|   IBIS model for TI xxx DSP
[IBIS Ver]   5.1
[Disclaimer]   Please be aware that in the absence of a written agreement
|   Texas Instruments(TI) assumes no liability for:
|   (1) The accuracy of the IBIS models provided to your company,
|   however, the IBIS model is compliant to industry standard
|   IQ Level 2a.  Refer to IBIS Quality Section below for
|   for full details.
|   (2) The proper functioning of these Models in your design
|   or for any resulting applications
|   (3) Infringement of patents, copyrights or intellectual
|   property rights resulting from your use of these
|   models.
|   TI provides IBIS Models as a service to our customers and
|   therefore reserves the right to limit distribution of the
|   Models.  The information is subject to change without notice.
[File Name]  sprm771.ibs
[File Rev]   0.1
|   -Initial version
|   -Updated Package model
[Date]   12 Aug 2021
[Source]   Texas Instruments Incorporated
[Copyright]   Property of Texas Instruments Incorporated.
|   Unauthorized reproduction and/or distribution is strictly.
|   prohibited.
|   This product is protected under copyright law and trade
|   secret law as an unpublished work.
|   Created 2012,(C) Copyright 1999-2012,
|   Texas Instruments Incorporated., All Rights Reserved.
|   These commodities are under the U.S. Government
|   distribution license control. As such,they are not to be
|   re-exported without the prior approval of the U.S.
|   Department of Commerce.
[Notes]
  ADC and DAC pins are marked as NC
  XTAL pins are marked as NC
|   Revision History
|   GERNERAL COMMENT: All IBIS Quality Notes below reflect latest release
|   and version of IBIS File
|   File passes ibischk6.0 with 0 errors and 125 warnings
|   Component AM263
[Component] AM263
[Manufacturer] Texas Instruments
[Package Model] AM263_pkg
[Package]
|   typ   min   max
R_pkg   0.11723   0.038857   0.22589
L_pkg   3.378e-9   1.178e-9   5.997e-9
C_pkg   6.073e-13   4.462e-13   1.294e-12
[Pin] Signal_name model_name | Buffer Name
E9   VDD   POWER
E11   VDD   POWER
F9   VDD   POWER
F11   VDD   POWER
G5   VDD   POWER
G6   VDD   POWER
G13   VDD   POWER
G14   VDD   POWER
K5   VDD   POWER
K6   VDD   POWER
K13   VDD   POWER
K14   VDD   POWER
N5   VDD   POWER
N6   VDD   POWER
N13   VDD   POWER
N14   VDD   POWER
R8   VDDA18   POWER
R11   VDDA18   POWER
R6   VDDA18_LDO   POWER
R4   VDDA18_OSC_PLL   POWER
P7   VDDA33   POWER
P9   VDDA33   POWER
P11   VDDA33   POWER
J15   VDDAR1   POWER
D10   VDDAR2   POWER
H3   VDDAR3   POWER
D6   VDDS18   POWER
E15   VDDS18   POWER
L4   VDDS18   POWER
N15   VDDS18   POWER
T3   VDDS18_LDO   POWER
D8   VDDS33   POWER
D12   VDDS33   POWER
H4   VDDS33   POWER
H15   VDDS33   POWER
L15   VDDS33   POWER
P4   VDDS33   POWER
R15   VDDS33   POWER
R9   VDD_F   POWER
J16   VNWA   POWER
N3   VPP   POWER
V15   ADC0_AIN0   NC
U15   ADC0_AIN1   NC
T14   ADC0_AIN2   NC
U14   ADC0_AIN3   NC
U13   ADC0_AIN4   NC
R14   ADC0_AIN5   NC
T11   ADC1_AIN0   NC
U11   ADC1_AIN1   NC
T12   ADC1_AIN2   NC
V12   ADC1_AIN3   NC
U12   ADC1_AIN4   NC
R12   ADC1_AIN5   NC
R10   ADC2_AIN0   NC
T10   ADC2_AIN1   NC
U10   ADC2_AIN2   NC
T9   ADC2_AIN3   NC
V9   ADC2_AIN4   NC
T8   ADC2_AIN5   NC
U7   ADC3_AIN0   NC
U8   ADC3_AIN1   NC
T7   ADC3_AIN2   NC
R7   ADC3_AIN3   NC
V8   ADC3_AIN4   NC
U9   ADC3_AIN5   NC
U6   ADC4_AIN0   NC
V5   ADC4_AIN1   NC
V4   ADC4_AIN2   NC
U5   ADC4_AIN3   NC
V3   ADC4_AIN4   NC
U4   ADC4_AIN5   NC
U16   ADC_CAL0   NC
T15   ADC_CAL1   NC
V14   ADC_VREFHI_G0   NC
V10   ADC_VREFHI_G1   NC
V6   ADC_VREFHI_G2   NC
V13   ADC_VREFLO_G0   NC
V11   ADC_VREFLO_G1   NC
V7   ADC_VREFLO_G2   NC
U3   ATESTV0   NC
V2   ATESTV1   NC
M2   CLKOUT0   bc1833dv40dcpbfbp18ll_ssdlv
T5   DAC_OUT   NC
T13   DAC_VREF0   NC
T6   DAC_VREF1   NC
B2   EPWM0_A   bc1833dv40dcpbfbp18ll_ssdlv
B1   EPWM0_B   bc1833dv40dcpbfbp18ll_ssdlv
D3   EPWM1_A   bc1833dv40dcpbfbp18ll_ssdlv
D2   EPWM1_B   bc1833dv40dcpbfbp18ll_ssdlv
C2   EPWM2_A   bc1833dv40dcpbfbp18ll_ssdlv
C1   EPWM2_B   bc1833dv40dcpbfbp18ll_ssdlv
E2   EPWM3_A   bc1833dv40dcpbfbp18ll_ssdlv
E3   EPWM3_B   bc1833dv40dcpbfbp18ll_ssdlv
D1   EPWM4_A   bc1833dv40dcpbfbp18ll_ssdlv
E4   EPWM4_B   bc1833dv40dcpbfbp18ll_ssdlv
F2   EPWM5_A   bc1833dv40dcpbfbp18ll_ssdlv
G2   EPWM5_B   bc1833dv40dcpbfbp18ll_ssdlv
E1   EPWM6_A   bc1833dv40dcpbfbp18ll_ssdlv
F3   EPWM6_B   bc1833dv40dcpbfbp18ll_ssdlv
F4   EPWM7_A   bc1833dv40dcpbfbp18ll_ssdlv
F1   EPWM7_B   bc1833dv40dcpbfbp18ll_ssdlv
G3   EPWM8_A   bc1833dv40dcpbfbp18ll_ssdlv
H2   EPWM8_B   bc1833dv40dcpbfbp18ll_ssdlv
G1   EPWM9_A   bc1833dv40dcpbfbp18ll_ssdlv
J2   EPWM9_B   bc1833dv40dcpbfbp18ll_ssdlv
G4   EPWM10_A   bc1833dv40dcpbfbp18ll_ssdlv
J3   EPWM10_B   bc1833dv40dcpbfbp18ll_ssdlv
H1   EPWM11_A   bc1833dv40dcpbfbp18ll_ssdlv
J1   EPWM11_B   bc1833dv40dcpbfbp18ll_ssdlv
K2   EPWM12_A   bc1833dv40dcpbfbp18ll_ssdlv
J4   EPWM12_B   bc1833dv40dcpbfbp18ll_ssdlv
K4   EPWM13_A   bc1833dv40dcpbfbp18ll_ssdlv
K3   EPWM13_B   bc1833dv40dcpbfbp18ll_ssdlv
V17   EPWM14_A   bc1833dv40dcpbfbp18ll_ssdlh
T16   EPWM14_B   bc1833dv40dcpbfbp18ll_ssdlh
P15   EPWM15_A   bc1833dv40dcpbfbp18ll_ssdlv
R16   EPWM15_B   bc1833dv40dcpbfbp18ll_ssdlv
B14   EQEP0_A   bc1833dv40dcpbfbp18ll_ssdlh
A14   EQEP0_B   bc1833dv40dcpbfbp18ll_ssdlh
D11   EQEP0_INDEX   bc1833dv40dcpbfbp18ll_ssdlh
C12   EQEP0_STROBE   bc1833dv40dcpbfbp18ll_ssdlh
P2   EXT_REFCLK0   bc1833dv40dcpbfbp18ll_ssdlv
A13   I2C0_SCL   bi2c1833dvfzp18_ssdlh
B13   I2C0_SDA   bi2c1833dvfzp18_ssdlh
D7   I2C1_SCL   bc1833dv40dcpbfbp18ll_ssdlh
C8   I2C1_SDA   bc1833dv40dcpbfbp18ll_ssdlh
A9   LIN1_RXD   bc1833dv40dcpbfbp18ll_ssdlh
B9   LIN1_TXD   bc1833dv40dcpbfbp18ll_ssdlh
B8   LIN2_RXD   bc1833dv40dcpbfbp18ll_ssdlh
A8   LIN2_TXD   bc1833dv40dcpbfbp18ll_ssdlh
M1   MCAN0_RX   bc1833dv40dcpbfbp18ll_ssdlv
L1   MCAN0_TX   bc1833dv40dcpbfbp18ll_ssdlv
L2   MCAN1_RX   bc1833dv40dcpbfbp18ll_ssdlv
K1   MCAN1_TX   bc1833dv40dcpbfbp18ll_ssdlv
A12   MCAN2_RX   bc1833dv40dcpbfbp18ll_ssdlh
B12   MCAN2_TX   bc1833dv40dcpbfbp18ll_ssdlh
M17   MDIO0_MDC   bc1833dv40dcpbfbp18ll_ssdlv
N16   MDIO0_MDIO   bc1833dv40dcpbfbp18ll_ssdlv
A5   MMC0_CD   bc1833dv40dcpbfbp18ll_ssdlh
B6   MMC0_CLK   bc1833dv40dcpbfbp18ll_ssdlh
A4   MMC0_CMD   bc1833dv40dcpbfbp18ll_ssdlh
B5   MMC0_D0   bc1833dv40dcpbfbp18ll_ssdlh
B4   MMC0_D1   bc1833dv40dcpbfbp18ll_ssdlh
A3   MMC0_D2   bc1833dv40dcpbfbp18ll_ssdlh
A2   MMC0_D3   bc1833dv40dcpbfbp18ll_ssdlh
C6   MMC0_WP   bc1833dv40dcpbfbp18ll_ssdlh
R2   PORZ   ihhv1833dvhyp18ll_ssdhv
L18   PR0_MDIO0_MDC   bc1833dv40dcpbfbp18ll_ssdlv
L17   PR0_MDIO0_MDIO   bc1833dv40dcpbfbp18ll_ssdlv
K17   PR0_PRU0_GPO0   bc1833dv40dcpbfbp18ll_ssdlv
K18   PR0_PRU0_GPO1   bc1833dv40dcpbfbp18ll_ssdlv
J18   PR0_PRU0_GPO2   bc1833dv40dcpbfbp18ll_ssdlv
J17   PR0_PRU0_GPO3   bc1833dv40dcpbfbp18ll_ssdlv
K16   PR0_PRU0_GPO4   bc1833dv40dcpbfbp18ll_ssdlv
G17   PR0_PRU0_GPO5   bc1833dv40dcpbfbp18ll_ssdlv
K15   PR0_PRU0_GPO6   bc1833dv40dcpbfbp18ll_ssdlv
G15   PR0_PRU0_GPO8   bc1833dv40dcpbfbp18ll_ssdlv
F17   PR0_PRU0_GPO9   bc1833dv40dcpbfbp18ll_ssdlv
G18   PR0_PRU0_GPO10   bc1833dv40dcpbfbp18ll_ssdlv
M16   PR0_PRU0_GPO11   bc1833dv40dcpbfbp18ll_ssdlv
M15   PR0_PRU0_GPO12   bc1833dv40dcpbfbp18ll_ssdlv
H17   PR0_PRU0_GPO13   bc1833dv40dcpbfbp18ll_ssdlv
H16   PR0_PRU0_GPO14   bc1833dv40dcpbfbp18ll_ssdlv
L16   PR0_PRU0_GPO15   bc1833dv40dcpbfbp18ll_ssdlv
H18   PR0_PRU0_GPO16   bc1833dv40dcpbfbp18ll_ssdlv
F18   PR0_PRU1_GPO0   bc1833dv40dcpbfbp18ll_ssdlv
G16   PR0_PRU1_GPO1   bc1833dv40dcpbfbp18ll_ssdlv
E17   PR0_PRU1_GPO2   bc1833dv40dcpbfbp18ll_ssdlv
E18   PR0_PRU1_GPO3   bc1833dv40dcpbfbp18ll_ssdlv
F16   PR0_PRU1_GPO4   bc1833dv40dcpbfbp18ll_ssdlv
F15   PR0_PRU1_GPO5   bc1833dv40dcpbfbp18ll_ssdlv
E16   PR0_PRU1_GPO6   bc1833dv40dcpbfbp18ll_ssdlv
D18   PR0_PRU1_GPO8   bc1833dv40dcpbfbp18ll_ssdlv
C18   PR0_PRU1_GPO9   bc1833dv40dcpbfbp18ll_ssdlv
D17   PR0_PRU1_GPO10   bc1833dv40dcpbfbp18ll_ssdlv
B18   PR0_PRU1_GPO11   bc1833dv40dcpbfbp18ll_ssdlv
B17   PR0_PRU1_GPO12   bc1833dv40dcpbfbp18ll_ssdlv
D16   PR0_PRU1_GPO13   bc1833dv40dcpbfbp18ll_ssdlv
C17   PR0_PRU1_GPO14   bc1833dv40dcpbfbp18ll_ssdlv
A17   PR0_PRU1_GPO15   bc1833dv40dcpbfbp18ll_ssdlv
C16   PR0_PRU1_GPO16   bc1833dv40dcpbfbp18ll_ssdlv
C15   PR0_PRU1_GPO18   bc1833dv40dcpbfbp18ll_ssdlv
D15   PR0_PRU1_GPO19   bc1833dv40dcpbfbp18ll_ssdlv
N2   QSPI0_CLK   bc1833dv40dcpbfbp18ll_ssdlv
P1   QSPI0_CSN0   bc1833dv40dcpbfbp18ll_ssdlv
R3   QSPI0_CSN1   bc1833dv40dcpbfbp18ll_ssdlv
N1   QSPI0_D0   bc1833dv40dcpbfbp18ll_ssdlv
N4   QSPI0_D1   bc1833dv40dcpbfbp18ll_ssdlv
M4   QSPI0_D2   bc1833dv40dcpbfbp18ll_ssdlv
P3   QSPI0_D3   bc1833dv40dcpbfbp18ll_ssdlv
U17   RGMII1_RD0   bc1833dv40dcpbfbp18ll_ssdlv
T17   RGMII1_RD1   bc1833dv40dcpbfbp18ll_ssdlv
U18   RGMII1_RD2   bc1833dv40dcpbfbp18ll_ssdlv
T18   RGMII1_RD3   bc1833dv40dcpbfbp18ll_ssdlv
R17   RGMII1_RXC   bc1833dv40dcpbfbp18ll_ssdlv
R18   RGMII1_RX_CTL   bc1833dv40dcpbfbp18ll_ssdlv
P16   RGMII1_TD0   bc1833dv40dcpbfbp18ll_ssdlv
P17   RGMII1_TD1   bc1833dv40dcpbfbp18ll_ssdlv
P18   RGMII1_TD2   bc1833dv40dcpbfbp18ll_ssdlv
N17   RGMII1_TD3   bc1833dv40dcpbfbp18ll_ssdlv
N18   RGMII1_TXC   bc1833dv40dcpbfbp18ll_ssdlv
M18   RGMII1_TX_CTL   bc1833dv40dcpbfbp18ll_ssdlv
D4   SAFETY_ERRORN   bc1833dv40dcpbfbp18ll_ssdlv
B16   SDFM0_CLK0   bc1833dv40dcpbfbp18ll_ssdlh
A16   SDFM0_CLK1   bc1833dv40dcpbfbp18ll_ssdlh
B15   SDFM0_CLK2   bc1833dv40dcpbfbp18ll_ssdlh
A15   SDFM0_CLK3   bc1833dv40dcpbfbp18ll_ssdlh
D14   SDFM0_D0   bc1833dv40dcpbfbp18ll_ssdlh
D13   SDFM0_D1   bc1833dv40dcpbfbp18ll_ssdlh
C13   SDFM0_D2   bc1833dv40dcpbfbp18ll_ssdlh
C14   SDFM0_D3   bc1833dv40dcpbfbp18ll_ssdlh
A11   SPI0_CLK   bc1833dv40dcpbfbp18ll_ssdlh
C11   SPI0_CS0   bc1833dv40dcpbfbp18ll_ssdlh
C10   SPI0_D0   bc1833dv40dcpbfbp18ll_ssdlh
B11   SPI0_D1   bc1833dv40dcpbfbp18ll_ssdlh
A10   SPI1_CLK   bc1833dv40dcpbfbp18ll_ssdlh
C9   SPI1_CS0   bc1833dv40dcpbfbp18ll_ssdlh
B10   SPI1_D0   bc1833dv40dcpbfbp18ll_ssdlh
D9   SPI1_D1   bc1833dv40dcpbfbp18ll_ssdlh
B3   TCK   iq1833dvtckpbfbp18ll_ssdhh
C5   TDI   bc1833dv40dcpbfbp18ll_ssdlh
C4   TDO   bc1833dv40dcpbfbp18ll_ssdlh
U1   TEMPCAL   NC
D5   TMS   bc1833dv40dcpbfbp18ll_ssdlh
B7   UART0_CTSN   bc1833dv40dcpbfbp18ll_ssdlh
C7   UART0_RTSN   bc1833dv40dcpbfbp18ll_ssdlh
A7   UART0_RXD   bc1833dv40dcpbfbp18ll_ssdlh
A6   UART0_TXD   bc1833dv40dcpbfbp18ll_ssdlh
L3   UART1_RXD   bc1833dv40dcpbfbp18ll_ssdlv
M3   UART1_TXD   bc1833dv40dcpbfbp18ll_ssdlv
T4   VDD_TEMP   NC
U2   VSYS_MON   NC
C3   WARMRSTN   bc1833dv40dcpbfbp18ll_od_fs_ssdlv
T1   XTAL_XI   NC
R1   XTAL_XO   NC
A1   VSS   GND
A18   VSS   GND
E5   VSS   GND
E6   VSS   GND
E7   VSS   GND
E8   VSS   GND
E10   VSS   GND
E12   VSS   GND
E13   VSS   GND
E14   VSS   GND
F5   VSS   GND
F6   VSS   GND
F7   VSS   GND
F8   VSS   GND
F10   VSS   GND
F12   VSS   GND
F13   VSS   GND
F14   VSS   GND
G7   VSS   GND
G8   VSS   GND
G9   VSS   GND
G10   VSS   GND
G11   VSS   GND
G12   VSS   GND
H5   VSS   GND
H6   VSS   GND
H7   VSS   GND
H8   VSS   GND
H9   VSS   GND
H10   VSS   GND
H11   VSS   GND
H12   VSS   GND
H13   VSS   GND
H14   VSS   GND
J5   VSS   GND
J6   VSS   GND
J7   VSS   GND
J8   VSS   GND
J9   VSS   GND
J10   VSS   GND
J11   VSS   GND
J12   VSS   GND
J13   VSS   GND
J14   VSS   GND
K7   VSS   GND
K8   VSS   GND
K9   VSS   GND
K10   VSS   GND
K11   VSS   GND
K12   VSS   GND
L5   VSS   GND
L6   VSS   GND
L7   VSS   GND
L8   VSS   GND
L9   VSS   GND
L10   VSS   GND
L11   VSS   GND
L12   VSS   GND
L13   VSS   GND
L14   VSS   GND
M5   VSS   GND
M6   VSS   GND
M7   VSS   GND
M8   VSS   GND
M9   VSS   GND
M10   VSS   GND
M11   VSS   GND
M12   VSS   GND
M13   VSS   GND
M14   VSS   GND
N7   VSS   GND
N8   VSS   GND
N9   VSS   GND
N10   VSS   GND
N11   VSS   GND
N12   VSS   GND
P5   VSS   GND
P13   VSS   GND
P14   VSS   GND
T2   VSS   GND
V18   VSS   GND
P6   VSSA   GND
P8   VSSA   GND
P10   VSSA   GND
P12   VSSA   GND
R5   VSSA   GND
R13   VSSA   GND
V1   VSSA   GND
V16   VSSA   GND
|   BC1833DV40DCPBFBP18LL_SSDLH
[Model Selector] bc1833dv40dcpbfbp18ll_ssdlh
|SC1 IS A SLEW RATE CONTROL PIN
|5% SUPPLY VARIATION MODES WITH 1.8V NOM SUPPLY
BC40D_H_PUPDOFF_5P_SC1_1P8  Cell operated at 1.8(nom)
|BC40D_H_PUPDOFF_5P_SC1_1P8; BUFFER WITH WEAK PULUP/PULLDOWN OFF AT 5% SUPPLY
|VARIATION WITH SC1=1 MEANING SLOW MODE OF OPERATION
BC40D_H_PD_ON_5P_!SC1_1P8  Cell operated at 1.8(nom)
|BC40D_H_PD_ON_5P_!SC1_1P8; BUFFER WITH WEAK_PULLDOWN_ON AT 5% SUPPLY
|VARIATION WITH SC1=0 MEANING FAST MODE OF OPERATION
BC40D_H_PD_ON_5P_SC1_1P8  Cell operated at 1.8(nom)
|BC40D_H_PD_ON_5P_SC1_1P8; BUFFER WITH WEAK_PULLDOWN_ON AT 5% SUPPLY
|VARIATION WITH SC1=1 MEANING SLOW MODE OF OPERATION
BC40D_H_PU_ON_5P_!SC1_1P8  Cell operated at 1.8(nom)
|BC40D_H_PU_ON_5P_!SC1_1P8; BUFFER WITH WEAK_PULLUP_ON AT 5% SUPPLY
|VARIATION WITH SC1=0 MEANING FAST MODE OF OPERATION
BC40D_H_PUPDOFF_5P_!SC1_1P8  Cell operated at 1.8(nom)
|BC40D_H_PUPDOFF_5P_!SC1_1P8; BUFFER WITH WEAK PULUP/PULLDOWN OFF AT 5% SUPPLY
|VARIATION WITH SC1=0 MEANING FAST MODE OF OPERATION
BC40D_H_PU_ON_5P_SC1_1P8  Cell operated at 1.8(nom)
|BC40D_H_PU_ON_5P_SC1_1P8; BUFFER WITH WEAK_PULLUP_ON AT 5% SUPPLY
|VARIATION WITH SC1=1 MEANING SLOW MODE OF OPERATION
|5% SUPPLY VARIATION MODES WITH 3.3V NOM SUPPLY
BC40D_H_PUPDOFF_5P_SC1_3P3  Cell operated at 3.3(nom)
|BC40D_H_PUPDOFF_5P_SC1_3P3; BUFFER WITH WEAK PULUP/PULLDOWN OFF AT 5% SUPPLY
|VARIATION WITH SC1=1 MEANING SLOW MODE OF OPERATION
BC40D_H_PD_ON_5P_!SC1_3P3  Cell operated at 3.3(nom)
|BC40D_H_PD_ON_5P_!SC1_3P3; BUFFER WITH WEAK_PULLDOWN_ON AT 5% SUPPLY
|VARIATION WITH SC1=0 MEANING FAST MODE OF OPERATION
BC40D_H_PD_ON_5P_SC1_3P3  Cell operated at 3.3(nom)
|BC40D_H_PD_ON_5P_SC1_3P3; BUFFER WITH WEAK_PULLDOWN_ON AT 5% SUPPLY
|VARIATION WITH SC1=1 MEANING SLOW MODE OF OPERATION
BC40D_H_PU_ON_5P_!SC1_3P3  Cell operated at 3.3(nom)
|BC40D_H_PU_ON_5P_!SC1_3P3; BUFFER WITH WEAK_PULLUP_ON AT 5% SUPPLY
|VARIATION WITH SC1=0 MEANING FAST MODE OF OPERATION
BC40D_H_PUPDOFF_5P_!SC1_3P3  Cell operated at 3.3(nom)
|BC40D_H_PUPDOFF_5P_!SC1_3P3; BUFFER WITH WEAK PULUP/PULLDOWN OFF AT 5% SUPPLY
|VARIATION WITH SC1=0 MEANING FAST MODE OF OPERATION
BC40D_H_PU_ON_5P_SC1_3P3  Cell operated at 3.3(nom)
|BC40D_H_PU_ON_5P_SC1_3P3; BUFFER WITH WEAK_PULLUP_ON AT 5% SUPPLY
|VARIATION WITH SC1=1 MEANING SLOW MODE OF OPERATION
| 10% SUPPLY VARIATION MODES WITH 1.8V NOM SUPPLY
BC40D_H_PUPDOFF_10P_SC1_1P8  Cell operated at 1.8(nom)
|BC40D_H_PUPDOFF_10P_SC1_1P8; BUFFER WITH WEAK PULUP/PULLDOWN OFF AT 10% SUPPLY
|VARIATION WITH SC1=1 MEANING SLOW MODE OF OPERATION
BC40D_H_PD_ON_10P_!SC1_1P8  Cell operated at 1.8(nom)
|BC40D_H_PD_ON_10P_!SC1_1P8; BUFFER WITH WEAK_PULLDOWN_ON AT 10% SUPPLY
|VARIATION WITH SC1=0 MEANING FAST MODE OF OPERATION
BC40D_H_PD_ON_10P_SC1_1P8  Cell operated at 1.8(nom)
|BC40D_H_PD_ON_10P_SC1_1P8; BUFFER WITH WEAK_PULLDOWN_ON AT 10% SUPPLY
|VARIATION WITH SC1=1 MEANING SLOW MODE OF OPERATION
BC40D_H_PU_ON_10P_!SC1_1P8  Cell operated at 1.8(nom)
|BC40D_H_PU_ON_10P_!SC1_1P8; BUFFER WITH WEAK_PULLUP_ON AT 10% SUPPLY
|VARIATION WITH SC1=0 MEANING FAST MODE OF OPERATION
BC40D_H_PUPDOFF_10P_!SC1_1P8  Cell operated at 1.8(nom)
|BC40D_H_PUPDOFF_10P_!SC1_1P8; BUFFER WITH WEAK PULUP/PULLDOWN OFF AT 10% SUPPLY
|VARIATION WITH SC1=0 MEANING FAST MODE OF OPERATION
BC40D_H_PU_ON_10P_SC1_1P8  Cell operated at 1.8(nom)
|BC40D_H_PU_ON_10P_SC1_1P8; BUFFER WITH WEAK_PULLUP_ON AT 10% SUPPLY
|VARIATION WITH SC1=1 MEANING SLOW MODE OF OPERATION
| 10% SUPPLY VARIATION MODES WITH 3.3V NOM SUPPLY
BC40D_H_PUPDOFF_10P_SC1_3P3  Cell operated at 3.3(nom)
|BC40D_H_PUPDOFF_10P_SC1_3P3; BUFFER WITH WEAK PULUP/PULLDOWN OFF AT 10% SUPPLY
|VARIATION WITH SC1=1 MEANING SLOW MODE OF OPERATION
BC40D_H_PD_ON_10P_!SC1_3P3  Cell operated at 3.3(nom)
|BC40D_H_PD_ON_10P_!SC1_3P3; BUFFER WITH WEAK_PULLDOWN_ON 10% SUPPLY
|VARIATION WITH SC1=0 MEANING FAST MODE OF OPERATION
BC40D_H_PD_ON_10P_SC1_3P3  Cell operated at 3.3(nom)
|BC40D_H_PD_ON_10P_SC1_3P3; BUFFER WITH WEAK_PULLDOWN_ON AT 10% SUPPLY
|VARIATION WITH SC1=1 MEANING SLOW MODE OF OPERATION
BC40D_H_PU_ON_10P_!SC1_3P3  Cell operated at 3.3(nom)
|BC40D_H_PU_ON_10P_!SC1_3P3; BUFFER WITH WEAK_PULLUP_ON AT 10% SUPPLY
|VARIATION WITH SC1=0 MEANING FAST MODE OF OPERATION
BC40D_H_PUPDOFF_10P_!SC1_3P3  Cell operated at 3.3(nom)
|BC40D_H_PUPDOFF_10P_!SC1_3P3; BUFFER WITH WEAK PULUP/PULLDOWN OFF AT 10% SUPPLY
|VARIATION WITH SC1=0 MEANING FAST MODE OF OPERATION
BC40D_H_PU_ON_10P_SC1_3P3  Cell operated at 3.3(nom)
|BC40D_H_PU_ON_10P_SC1_3P3; BUFFER WITH WEAK_PULLUP_ON AT 10% SUPPLY
|VARIATION WITH SC1=1 MEANING SLOW MODE OF OPERATION
|   BC1833DV40DCPBFBP18LL_SSDLV
[Model Selector] bc1833dv40dcpbfbp18ll_ssdlv
|SC1 IS A SLEW RATE CONTROL PIN
|5% SUPPLY VARIATION MODES WITH 1.8V NOM SUPPLY
BC40D_V_PUPDOFF_5P_SC1_1P8  Cell operated at 1.8(nom)
|BC40D_V_PUPDOFF_5P_SC1_1P8; BUFFER WITH WEAK PULUP/PULLDOWN OFF AT 5% SUPPLY
|VARIATION WITH SC1=1 MEANING SLOW MODE OF OPERATION
BC40D_V_PD_ON_5P_!SC1_1P8  Cell operated at 1.8(nom)
|BC40D_V_PD_ON_5P_!SC1_1P8; BUFFER WITH WEAK_PULLDOWN_ON AT 5% SUPPLY
|VARIATION WITH SC1=0 MEANING FAST MODE OF OPERATION
BC40D_V_PD_ON_5P_SC1_1P8  Cell operated at 1.8(nom)
|BC40D_V_PD_ON_5P_SC1_1P8; BUFFER WITH WEAK_PULLDOWN_ON AT 5% SUPPLY
|VARIATION WITH SC1=1 MEANING SLOW MODE OF OPERATION
BC40D_V_PU_ON_5P_!SC1_1P8  Cell operated at 1.8(nom)
|BC40D_V_PU_ON_5P_!SC1_1P8; BUFFER WITH WEAK_PULLUP_ON AT 5% SUPPLY
|VARIATION WITH SC1=0 MEANING FAST MODE OF OPERATION
BC40D_V_PUPDOFF_5P_!SC1_1P8  Cell operated at 1.8(nom)
|BC40D_V_PUPDOFF_5P_!SC1_1P8; BUFFER WITH WEAK PULUP/PULLDOWN OFF AT 5% SUPPLY
|VARIATION WITH SC1=0 MEANING FAST MODE OF OPERATION
BC40D_V_PU_ON_5P_SC1_1P8  Cell operated at 1.8(nom)
|BC40D_V_PU_ON_5P_SC1_1P8; BUFFER WITH WEAK_PULLUP_ON AT 5% SUPPLY
|VARIATION WITH SC1=1 MEANING SLOW MODE OF OPERATION
|5% SUPPLY VARIATION MODES WITH 3.3V NOM SUPPLY
BC40D_V_PUPDOFF_5P_SC1_3P3  Cell operated at 3.3(nom)
|BC40D_V_PUPDOFF_5P_SC1_3P3; BUFFER WITH WEAK PULUP/PULLDOWN OFF AT 5% SUPPLY
|VARIATION WITH SC1=1 MEANING SLOW MODE OF OPERATION
BC40D_V_PD_ON_5P_!SC1_3P3  Cell operated at 3.3(nom)
|BC40D_V_PD_ON_5P_!SC1_3P3; BUFFER WITH WEAK_PULLDOWN_ON AT 5% SUPPLY
|VARIATION WITH SC1=0 MEANING FAST MODE OF OPERATION
BC40D_V_PD_ON_5P_SC1_3P3  Cell operated at 3.3(nom)
|BC40D_V_PD_ON_5P_SC1_3P3; BUFFER WITH WEAK_PULLDOWN_ON AT 5% SUPPLY
|VARIATION WITH SC1=1 MEANING SLOW MODE OF OPERATION
BC40D_V_PU_ON_5P_!SC1_3P3  Cell operated at 3.3(nom)
|BC40D_V_PU_ON_5P_!SC1_3P3; BUFFER WITH WEAK_PULLUP_ON AT 5% SUPPLY
|VARIATION WITH SC1=0 MEANING FAST MODE OF OPERATION
BC40D_V_PUPDOFF_5P_!SC1_3P3  Cell operated at 3.3(nom)
|BC40D_V_PUPDOFF_5P_!SC1_3P3; BUFFER WITH WEAK PULUP/PULLDOWN OFF AT 5% SUPPLY
|VARIATION WITH SC1=0 MEANING FAST MODE OF OPERATION
BC40D_V_PU_ON_5P_SC1_3P3  Cell operated at 3.3(nom)
|BC40D_V_PU_ON_5P_SC1_3P3; BUFFER WITH WEAK_PULLUP_ON AT 5% SUPPLY
|VARIATION WITH SC1=1 MEANING SLOW MODE OF OPERATION
| 10% SUPPLY VARIATION MODES WITH 1.8V NOM SUPPLY
BC40D_V_PUPDOFF_10P_SC1_1P8  Cell operated at 1.8(nom)
|BC40D_V_PUPDOFF_10P_SC1_1P8; BUFFER WITH WEAK PULUP/PULLDOWN OFF AT 10% SUPPLY
|VARIATION WITH SC1=1 MEANING SLOW MODE OF OPERATION
BC40D_V_PD_ON_10P_!SC1_1P8  Cell operated at 1.8(nom)
|BC40D_V_PD_ON_10P_!SC1_1P8; BUFFER WITH WEAK_PULLDOWN_ON AT 10% SUPPLY
|VARIATION WITH SC1=0 MEANING FAST MODE OF OPERATION
BC40D_V_PD_ON_10P_SC1_1P8  Cell operated at 1.8(nom)
|BC40D_V_PD_ON_10P_SC1_1P8; BUFFER WITH WEAK_PULLDOWN_ON AT 10% SUPPLY
|VARIATION WITH SC1=1 MEANING SLOW MODE OF OPERATION
BC40D_V_PU_ON_10P_!SC1_1P8  Cell operated at 1.8(nom)
|BC40D_V_PU_ON_10P_!SC1_1P8; BUFFER WITH WEAK_PULLUP_ON AT 10% SUPPLY
|VARIATION WITH SC1=0 MEANING FAST MODE OF OPERATION
BC40D_V_PUPDOFF_10P_!SC1_1P8  Cell operated at 1.8(nom)
|BC40D_V_PUPDOFF_10P_!SC1_1P8; BUFFER WITH WEAK PULUP/PULLDOWN OFF AT 10% SUPPLY
|VARIATION WITH SC1=0 MEANING FAST MODE OF OPERATION
BC40D_V_PU_ON_10P_SC1_1P8  Cell operated at 1.8(nom)
|BC40D_V_PU_ON_10P_SC1_1P8; BUFFER WITH WEAK_PULLUP_ON AT 10% SUPPLY
|VARIATION WITH SC1=1 MEANING SLOW MODE OF OPERATION
| 10% SUPPLY VARIATION MODES WITH 3.3V NOM SUPPLY
BC40D_V_PUPDOFF_10P_SC1_3P3  Cell operated at 3.3(nom)
|BC40D_V_PUPDOFF_10P_SC1_3P3; BUFFER WITH WEAK PULUP/PULLDOWN OFF AT 10% SUPPLY
|VARIATION WITH SC1=1 MEANING SLOW MODE OF OPERATION
BC40D_V_PD_ON_10P_!SC1_3P3  Cell operated at 3.3(nom)
|BC40D_V_PD_ON_10P_!SC1_3P3; BUFFER WITH WEAK_PULLDOWN_ON 10% SUPPLY
|VARIATION WITH SC1=0 MEANING FAST MODE OF OPERATION
BC40D_V_PD_ON_10P_SC1_3P3  Cell operated at 3.3(nom)
|BC40D_V_PD_ON_10P_SC1_3P3; BUFFER WITH WEAK_PULLDOWN_ON AT 10% SUPPLY
|VARIATION WITH SC1=1 MEANING SLOW MODE OF OPERATION
BC40D_V_PU_ON_10P_!SC1_3P3  Cell operated at 3.3(nom)
|BC40D_V_PU_ON_10P_!SC1_3P3; BUFFER WITH WEAK_PULLUP_ON AT 10% SUPPLY
|VARIATION WITH SC1=0 MEANING FAST MODE OF OPERATION
BC40D_V_PUPDOFF_10P_!SC1_3P3  Cell operated at 3.3(nom)
|BC40D_V_PUPDOFF_10P_!SC1_3P3; BUFFER WITH WEAK PULUP/PULLDOWN OFF AT 10% SUPPLY
|VARIATION WITH SC1=0 MEANING FAST MODE OF OPERATION
BC40D_V_PU_ON_10P_SC1_3P3  Cell operated at 3.3(nom)
|BC40D_V_PU_ON_10P_SC1_3P3; BUFFER WITH WEAK_PULLUP_ON AT 10% SUPPLY
|VARIATION WITH SC1=1 MEANING SLOW MODE OF OPERATION
|   BI2C1833DVFZP18_SSDLH
[Model Selector] bi2c1833dvfzp18_ssdlh
BI2C1833_NORAML_5P_1P8  Cell operated at 1.8(nom)
|BI2C1833_NORAML_5P_1P8; I2C MODE AT 1.8V WITH 5% SUPPLY VARIATION
BI2C1833_NORAML_5P_3P3  Cell operated at 3.3(nom)
|BI2C1833_NORAML_5P_3P3; I2C MODE AT 3.3V WITH 5% SUPPLY VARIATION
BI2C1833_NORAML_10P_1P8  Cell operated at 1.8(nom)
|BI2C1833_NORAML_10P_1P8; I2C MODE AT 1.8V WITH 10% SUPPLY VARIATION
BI2C1833_NORAML_10P_3P3  Cell operated at 3.3(nom)
|BI2C1833_NORAML_10P_3P3; I2C MODE AT 3.3V WITH 10% SUPPLY VARIATION
|   IHHV1833DVHYP18LL_SSDHV
[Model Selector] ihhv1833dvhyp18ll_ssdhv
IHHV_NORAML_5P_1P8  Cell operated at 1.8(nom)
|IHHV_NORAML_5P_1P8; NORMAL MODE AT 1.8V WITH 5% SUPPLY VARIATION
IHHV_NORAML_5P_3P3  Cell operated at 3.3(nom)
|IHHV_NORAML_5P_3P3; NORMAL MODE AT 3.3V WITH 5% SUPPLY VARIATION
IHHV_NORAML_10P_1P8  Cell operated at 1.8(nom)
|IHHV_NORAML_10P_1P8; NORMAL MODE AT 1.8V WITH 10% SUPPLY VARIATION
IHHV_NORAML_10P_3P3  Cell operated at 3.3(nom)
|IHHV_NORAML_10P_3P3; NORMAL MODE AT 3.3V WITH 10% SUPPLY VARIATION
|   BC1833DV40DCPBFBP18LL_OD_FS_SSDLV
[Model Selector] bc1833dv40dcpbfbp18ll_od_fs_ssdlv
|SC1 IS A SLEW RATE CONTROL PIN
|5% SUPPLY VARIATION MODES WITH 1.8V NOM SUPPLY
BC40D_V_PUPDOFF_5P_SC1_1P8  Cell operated at 1.8(nom)
|BC40D_V_PUPDOFF_5P_SC1_1P8; BUFFER WITH WEAK PULUP/PULLDOWN OFF AT 5% SUPPLY
|VARIATION WITH SC1=1 MEANING SLOW MODE OF OPERATION
BC40D_V_PD_ON_5P_!SC1_1P8  Cell operated at 1.8(nom)
|BC40D_V_PD_ON_5P_!SC1_1P8; BUFFER WITH WEAK_PULLDOWN_ON AT 5% SUPPLY
|VARIATION WITH SC1=0 MEANING FAST MODE OF OPERATION
BC40D_V_PD_ON_5P_SC1_1P8  Cell operated at 1.8(nom)
|BC40D_V_PD_ON_5P_SC1_1P8; BUFFER WITH WEAK_PULLDOWN_ON AT 5% SUPPLY
|VARIATION WITH SC1=1 MEANING SLOW MODE OF OPERATION
BC40D_V_PU_ON_5P_!SC1_1P8  Cell operated at 1.8(nom)
|BC40D_V_PU_ON_5P_!SC1_1P8; BUFFER WITH WEAK_PULLUP_ON AT 5% SUPPLY
|VARIATION WITH SC1=0 MEANING FAST MODE OF OPERATION
BC40D_V_PUPDOFF_5P_!SC1_1P8  Cell operated at 1.8(nom)
|BC40D_V_PUPDOFF_5P_!SC1_1P8; BUFFER WITH WEAK PULUP/PULLDOWN OFF AT 5% SUPPLY
|VARIATION WITH SC1=0 MEANING FAST MODE OF OPERATION
BC40D_V_PU_ON_5P_SC1_1P8  Cell operated at 1.8(nom)
|BC40D_V_PU_ON_5P_SC1_1P8; BUFFER WITH WEAK_PULLUP_ON AT 5% SUPPLY
|VARIATION WITH SC1=1 MEANING SLOW MODE OF OPERATION
|5% SUPPLY VARIATION MODES WITH 3.3V NOM SUPPLY
BC40D_V_PUPDOFF_5P_SC1_3P3  Cell operated at 3.3(nom)
|BC40D_V_PUPDOFF_5P_SC1_3P3; BUFFER WITH WEAK PULUP/PULLDOWN OFF AT 5% SUPPLY
|VARIATION WITH SC1=1 MEANING SLOW MODE OF OPERATION
BC40D_V_PD_ON_5P_!SC1_3P3  Cell operated at 3.3(nom)
|BC40D_V_PD_ON_5P_!SC1_3P3; BUFFER WITH WEAK_PULLDOWN_ON AT 5% SUPPLY
|VARIATION WITH SC1=0 MEANING FAST MODE OF OPERATION
BC40D_V_PD_ON_5P_SC1_3P3  Cell operated at 3.3(nom)
|BC40D_V_PD_ON_5P_SC1_3P3; BUFFER WITH WEAK_PULLDOWN_ON AT 5% SUPPLY
|VARIATION WITH SC1=1 MEANING SLOW MODE OF OPERATION
BC40D_V_PU_ON_5P_!SC1_3P3  Cell operated at 3.3(nom)
|BC40D_V_PU_ON_5P_!SC1_3P3; BUFFER WITH WEAK_PULLUP_ON AT 5% SUPPLY
|VARIATION WITH SC1=0 MEANING FAST MODE OF OPERATION
BC40D_V_PUPDOFF_5P_!SC1_3P3  Cell operated at 3.3(nom)
|BC40D_V_PUPDOFF_5P_!SC1_3P3; BUFFER WITH WEAK PULUP/PULLDOWN OFF AT 5% SUPPLY
|VARIATION WITH SC1=0 MEANING FAST MODE OF OPERATION
BC40D_V_PU_ON_5P_SC1_3P3  Cell operated at 3.3(nom)
|BC40D_V_PU_ON_5P_SC1_3P3; BUFFER WITH WEAK_PULLUP_ON AT 5% SUPPLY
|VARIATION WITH SC1=1 MEANING SLOW MODE OF OPERATION
| 10% SUPPLY VARIATION MODES WITH 1.8V NOM SUPPLY
BC40D_V_PUPDOFF_10P_SC1_1P8  Cell operated at 1.8(nom)
|BC40D_V_PUPDOFF_10P_SC1_1P8; BUFFER WITH WEAK PULUP/PULLDOWN OFF AT 10% SUPPLY
|VARIATION WITH SC1=1 MEANING SLOW MODE OF OPERATION
BC40D_V_PD_ON_10P_!SC1_1P8  Cell operated at 1.8(nom)
|BC40D_V_PD_ON_10P_!SC1_1P8; BUFFER WITH WEAK_PULLDOWN_ON AT 10% SUPPLY
|VARIATION WITH SC1=0 MEANING FAST MODE OF OPERATION
BC40D_V_PD_ON_10P_SC1_1P8  Cell operated at 1.8(nom)
|BC40D_V_PD_ON_10P_SC1_1P8; BUFFER WITH WEAK_PULLDOWN_ON AT 10% SUPPLY
|VARIATION WITH SC1=1 MEANING SLOW MODE OF OPERATION
BC40D_V_PU_ON_10P_!SC1_1P8  Cell operated at 1.8(nom)
|BC40D_V_PU_ON_10P_!SC1_1P8; BUFFER WITH WEAK_PULLUP_ON AT 10% SUPPLY
|VARIATION WITH SC1=0 MEANING FAST MODE OF OPERATION
BC40D_V_PUPDOFF_10P_!SC1_1P8  Cell operated at 1.8(nom)
|BC40D_V_PUPDOFF_10P_!SC1_1P8; BUFFER WITH WEAK PULUP/PULLDOWN OFF AT 10% SUPPLY
|VARIATION WITH SC1=0 MEANING FAST MODE OF OPERATION
BC40D_V_PU_ON_10P_SC1_1P8  Cell operated at 1.8(nom)
|BC40D_V_PU_ON_10P_SC1_1P8; BUFFER WITH WEAK_PULLUP_ON AT 10% SUPPLY
|VARIATION WITH SC1=1 MEANING SLOW MODE OF OPERATION
| 10% SUPPLY VARIATION MODES WITH 3.3V NOM SUPPLY
BC40D_V_PUPDOFF_10P_SC1_3P3  Cell operated at 3.3(nom)
|BC40D_V_PUPDOFF_10P_SC1_3P3; BUFFER WITH WEAK PULUP/PULLDOWN OFF AT 10% SUPPLY
|VARIATION WITH SC1=1 MEANING SLOW MODE OF OPERATION
BC40D_V_PD_ON_10P_!SC1_3P3  Cell operated at 3.3(nom)
|BC40D_V_PD_ON_10P_!SC1_3P3; BUFFER WITH WEAK_PULLDOWN_ON 10% SUPPLY
|VARIATION WITH SC1=0 MEANING FAST MODE OF OPERATION
BC40D_V_PD_ON_10P_SC1_3P3  Cell operated at 3.3(nom)
|BC40D_V_PD_ON_10P_SC1_3P3; BUFFER WITH WEAK_PULLDOWN_ON AT 10% SUPPLY
|VARIATION WITH SC1=1 MEANING SLOW MODE OF OPERATION
BC40D_V_PU_ON_10P_!SC1_3P3  Cell operated at 3.3(nom)
|BC40D_V_PU_ON_10P_!SC1_3P3; BUFFER WITH WEAK_PULLUP_ON AT 10% SUPPLY
|VARIATION WITH SC1=0 MEANING FAST MODE OF OPERATION
BC40D_V_PUPDOFF_10P_!SC1_3P3  Cell operated at 3.3(nom)
|BC40D_V_PUPDOFF_10P_!SC1_3P3; BUFFER WITH WEAK PULUP/PULLDOWN OFF AT 10% SUPPLY
|VARIATION WITH SC1=0 MEANING FAST MODE OF OPERATION
BC40D_V_PU_ON_10P_SC1_3P3  Cell operated at 3.3(nom)
|BC40D_V_PU_ON_10P_SC1_3P3; BUFFER WITH WEAK_PULLUP_ON AT 10% SUPPLY
|VARIATION WITH SC1=1 MEANING SLOW MODE OF OPERATION
|   IQ1833DVTCKPBFBP18LL_SSDHH
[Model Selector] iq1833dvtckpbfbp18ll_ssdhh
|5% SUPPLY VARIATION MODES WITH 1.8V NOM SUPPLY
IQ_SSDHH_PD_ON_5P_1P8  Cell operated at 1.8(nom)
|IQ_SSDHH_PD_ON_5P_1P8; BUFFER WITH WEAK_PULLDOWN_ON AT 5% SUPPLY VARIATION
IQ_SSDHH_PU_ON_5P_1P8  Cell operated at 1.8(nom)
|IQ_SSDHH_PU_ON_5P_1P8; BUFFER WITH WEAK_PULLUP_ON AT 5% SUPPLY VARIATION
IQ_SSDHH_PUPDOFF_5P_1P8  Cell operated at 1.8(nom)
|IQ_SSDHH_PUPDOFF_5P_1P8; BUFFER WITH WEAK PUPD OFF AT 5% SUPPLY VARIATION
|5% SUPPLY VARIATION MODES WITH 3.3V NOM SUPPLY
IQ_SSDHH_PD_ON_5P_3P3  Cell operated at 3.3(nom)
|IQ_SSDHH_PD_ON_5P_3P3; BUFFER WITH WEAK_PULLDOWN_ON AT 5% SUPPLY VARIATION
IQ_SSDHH_PU_ON_5P_3P3  Cell operated at 3.3(nom)
|IQ_SSDHH_PU_ON_5P_3P3; BUFFER WITH WEAK_PULLUP_ON AT 5% SUPPLY VARIATION
IQ_SSDHH_PUPDOFF_5P_3P3  Cell operated at 3.3(nom)
|IQ_SSDHH_PUPDOFF_5P_3P3; BUFFER WITH WEAK PUPD OFF AT 5% SUPPLY VARIATION
|10% SUPPLY VARIATION MODES WITH 1.8V NOM SUPPLY
IQ_SSDHH_PD_ON_10P_1P8  Cell operated at 1.8(nom)
|IQ_SSDHH_PD_ON_10P_1P8; BUFFER WITH WEAK_PULLDOWN_ON AT 10% SUPPLY VARIATION
IQ_SSDHH_PU_ON_10P_1P8  Cell operated at 1.8(nom)
|IQ_SSDHH_PU_ON_10P_1P8; BUFFER WITH WEAK_PULLUP_ON AT 10% SUPPLY VARIATION
IQ_SSDHH_PUPDOFF_10P_1P8  Cell operated at 1.8(nom)
|IQ_SSDHH_PUPDOFF_10P_1P8; BUFFER WITH WEAK PUPD OFF AT 10% SUPPLY VARIATION
|10% SUPPLY VARIATION MODES WITH 3.3V NOM SUPPLY
IQ_SSDHH_PD_ON_10P_3P3  Cell operated at 3.3(nom)
|IQ_SSDHH_PD_ON_10P_3P3; BUFFER WITH WEAK_PULLDOWN_ON  AT 10% SUPPLY VARIATION
IQ_SSDHH_PU_ON_10P_3P3  Cell operated at 3.3(nom)
|IQ_SSDHH_PU_ON_10P_3P3; BUFFER WITH WEAK_PULLUP_ON AT 10% SUPPLY VARIATION
IQ_SSDHH_PUPDOFF_10P_3P3  Cell operated at 3.3(nom)
|   Package Model
[Define Package Model]   AM263_pkg
[Manufacturer]   name 1
[OEM]   name 2
[Description]   208-pin Package
|[Number of Sections]   1
[Number of Pins]   208
[Pin Numbers]
|[Pin Name]  Net Number   Net Name   Net's All Pins
E9   | 1   VDD   E9
   |E11
   |F9
   |F11
   |G5
   |G6
   |G13
   |G14
   |K5
   |K6
   |K13
   |K14
   |N5
   |N6
   |N13
   |N14
R8   | 2   VDDA18   R8
   |R11
R6   | 3   VDDA18_LDO   R6
R4   | 4   VDDA18_OSC_PLL   R4
P7   | 5   VDDA33   P7
   |P9
   |P11
J15   | 6   VDDAR1   J15
D10   | 7   VDDAR2   D10
H3   | 8   VDDAR3   H3
D6   | 9   VDDS18   D6
   |E15
   |L4
   |N15
T3   | 10   VDDS18_LDO   T3
D8   | 11   VDDS33   D8
   |D12
   |H4
   |H15
   |L15
   |P4
   |R15
R9   | 12   VDD_F   R9
J16   | 13   VNWA   J16
N3   | 14   VPP   N3
V15   | 15   ADC0_AIN0   V15
U15   | 16   ADC0_AIN1   U15
T14   | 17   ADC0_AIN2   T14
U14   | 18   ADC0_AIN3   U14
U13   | 19   ADC0_AIN4   U13
R14   | 20   ADC0_AIN5   R14
T11   | 21   ADC1_AIN0   T11
U11   | 22   ADC1_AIN1   U11
T12   | 23   ADC1_AIN2   T12
V12   | 24   ADC1_AIN3   V12
U12   | 25   ADC1_AIN4   U12
R12   | 26   ADC1_AIN5   R12
R10   | 27   ADC2_AIN0   R10
T10   | 28   ADC2_AIN1   T10
U10   | 29   ADC2_AIN2   U10
T9   | 30   ADC2_AIN3   T9
V9   | 31   ADC2_AIN4   V9
T8   | 32   ADC2_AIN5   T8
U7   | 33   ADC3_AIN0   U7
U8   | 34   ADC3_AIN1   U8
T7   | 35   ADC3_AIN2   T7
R7   | 36   ADC3_AIN3   R7
V8   | 37   ADC3_AIN4   V8
U9   | 38   ADC3_AIN5   U9
U6   | 39   ADC4_AIN0   U6
V5   | 40   ADC4_AIN1   V5
V4   | 41   ADC4_AIN2   V4
U5   | 42   ADC4_AIN3   U5
V3   | 43   ADC4_AIN4   V3
U4   | 44   ADC4_AIN5   U4
U16   | 45   ADC_CAL0   U16
T15   | 46   ADC_CAL1   T15
V14   | 47   ADC_VREFHI_G0   V14
V10   | 48   ADC_VREFHI_G1   V10
V6   | 49   ADC_VREFHI_G2   V6
V13   | 50   ADC_VREFLO_G0   V13
V11   | 51   ADC_VREFLO_G1   V11
V7   | 52   ADC_VREFLO_G2   V7
U3   | 53   ATESTV0   U3
V2   | 54   ATESTV1   V2
M2   | 55   CLKOUT0   M2
T5   | 56   DAC_OUT   T5
T13   | 57   DAC_VREF0   T13
T6   | 58   DAC_VREF1   T6
B2   | 59   EPWM0_A   B2
B1   | 60   EPWM0_B   B1
D3   | 61   EPWM1_A   D3
D2   | 62   EPWM1_B   D2
C2   | 63   EPWM2_A   C2
C1   | 64   EPWM2_B   C1
E2   | 65   EPWM3_A   E2
E3   | 66   EPWM3_B   E3
D1   | 67   EPWM4_A   D1
E4   | 68   EPWM4_B   E4
F2   | 69   EPWM5_A   F2
G2   | 70   EPWM5_B   G2
E1   | 71   EPWM6_A   E1
F3   | 72   EPWM6_B   F3
F4   | 73   EPWM7_A   F4
F1   | 74   EPWM7_B   F1
G3   | 75   EPWM8_A   G3
H2   | 76   EPWM8_B   H2
G1   | 77   EPWM9_A   G1
J2   | 78   EPWM9_B   J2
G4   | 79   EPWM10_A   G4
J3   | 80   EPWM10_B   J3
H1   | 81   EPWM11_A   H1
J1   | 82   EPWM11_B   J1
K2   | 83   EPWM12_A   K2
J4   | 84   EPWM12_B   J4
K4   | 85   EPWM13_A   K4
K3   | 86   EPWM13_B   K3
V17   | 87   EPWM14_A   V17
T16   | 88   EPWM14_B   T16
P15   | 89   EPWM15_A   P15
R16   | 90   EPWM15_B   R16
B14   | 91   EQEP0_A   B14
A14   | 92   EQEP0_B   A14
D11   | 93   EQEP0_INDEX   D11
C12   | 94   EQEP0_STROBE   C12
P2   | 95   EXT_REFCLK0   P2
A13   | 96   I2C0_SCL   A13
B13   | 97   I2C0_SDA   B13
D7   | 98   I2C1_SCL   D7
C8   | 99   I2C1_SDA   C8
A9   | 100   LIN1_RXD   A9
B9   | 101   LIN1_TXD   B9
B8   | 102   LIN2_RXD   B8
A8   | 103   LIN2_TXD   A8
M1   | 104   MCAN0_RX   M1
L1   | 105   MCAN0_TX   L1
L2   | 106   MCAN1_RX   L2
K1   | 107   MCAN1_TX   K1
A12   | 108   MCAN2_RX   A12
B12   | 109   MCAN2_TX   B12
M17   | 110   MDIO0_MDC   M17
N16   | 111   MDIO0_MDIO   N16
A5   | 112   MMC0_CD   A5
B6   | 113   MMC0_CLK   B6
A4   | 114   MMC0_CMD   A4
B5   | 115   MMC0_D0   B5
B4   | 116   MMC0_D1   B4
A3   | 117   MMC0_D2   A3
A2   | 118   MMC0_D3   A2
C6   | 119   MMC0_WP   C6
R2   | 120   PORZ   R2
L18   | 121   PR0_MDIO0_MDC   L18
L17   | 122   PR0_MDIO0_MDIO   L17
K17   | 123   PR0_PRU0_GPO0   K17
K18   | 124   PR0_PRU0_GPO1   K18
J18   | 125   PR0_PRU0_GPO2   J18
J17   | 126   PR0_PRU0_GPO3   J17
K16   | 127   PR0_PRU0_GPO4   K16
G17   | 128   PR0_PRU0_GPO5   G17
K15   | 129   PR0_PRU0_GPO6   K15
G15   | 130   PR0_PRU0_GPO8   G15
F17   | 131   PR0_PRU0_GPO9   F17
G18   | 132   PR0_PRU0_GPO10   G18
M16   | 133   PR0_PRU0_GPO11   M16
M15   | 134   PR0_PRU0_GPO12   M15
H17   | 135   PR0_PRU0_GPO13   H17
H16   | 136   PR0_PRU0_GPO14   H16
L16   | 137   PR0_PRU0_GPO15   L16
H18   | 138   PR0_PRU0_GPO16   H18
F18   | 139   PR0_PRU1_GPO0   F18
G16   | 140   PR0_PRU1_GPO1   G16
E17   | 141   PR0_PRU1_GPO2   E17
E18   | 142   PR0_PRU1_GPO3   E18
F16   | 143   PR0_PRU1_GPO4   F16
F15   | 144   PR0_PRU1_GPO5   F15
E16   | 145   PR0_PRU1_GPO6   E16
D18   | 146   PR0_PRU1_GPO8   D18
C18   | 147   PR0_PRU1_GPO9   C18
D17   | 148   PR0_PRU1_GPO10   D17
B18   | 149   PR0_PRU1_GPO11   B18
B17   | 150   PR0_PRU1_GPO12   B17
D16   | 151   PR0_PRU1_GPO13   D16
C17   | 152   PR0_PRU1_GPO14   C17
A17   | 153   PR0_PRU1_GPO15   A17
C16   | 154   PR0_PRU1_GPO16   C16
C15   | 155   PR0_PRU1_GPO18   C15
D15   | 156   PR0_PRU1_GPO19   D15
N2   | 157   QSPI0_CLK   N2
P1   | 158   QSPI0_CSN0   P1
R3   | 159   QSPI0_CSN1   R3
N1   | 160   QSPI0_D0   N1
N4   | 161   QSPI0_D1   N4
M4   | 162   QSPI0_D2   M4
P3   | 163   QSPI0_D3   P3
U17   | 164   RGMII1_RD0   U17
T17   | 165   RGMII1_RD1   T17
U18   | 166   RGMII1_RD2   U18
T18   | 167   RGMII1_RD3   T18
R17   | 168   RGMII1_RXC   R17
R18   | 169   RGMII1_RX_CTL   R18
P16   | 170   RGMII1_TD0   P16
P17   | 171   RGMII1_TD1   P17
P18   | 172   RGMII1_TD2   P18
N17   | 173   RGMII1_TD3   N17
N18   | 174   RGMII1_TXC   N18
M18   | 175   RGMII1_TX_CTL   M18
D4   | 176   SAFETY_ERRORN   D4
B16   | 177   SDFM0_CLK0   B16
A16   | 178   SDFM0_CLK1   A16
B15   | 179   SDFM0_CLK2   B15
A15   | 180   SDFM0_CLK3   A15
D14   | 181   SDFM0_D0   D14
D13   | 182   SDFM0_D1   D13
C13   | 183   SDFM0_D2   C13
C14   | 184   SDFM0_D3   C14
A11   | 185   SPI0_CLK   A11
C11   | 186   SPI0_CS0   C11
C10   | 187   SPI0_D0   C10
B11   | 188   SPI0_D1   B11
A10   | 189   SPI1_CLK   A10
C9   | 190   SPI1_CS0   C9
B10   | 191   SPI1_D0   B10
D9   | 192   SPI1_D1   D9
B3   | 193   TCK   B3
C5   | 194   TDI   C5
C4   | 195   TDO   C4
U1   | 196   TEMPCAL   U1
D5   | 197   TMS   D5
B7   | 198   UART0_CTSN   B7
C7   | 199   UART0_RTSN   C7
A7   | 200   UART0_RXD   A7
A6   | 201   UART0_TXD   A6
L3   | 202   UART1_RXD   L3
M3   | 203   UART1_TXD   M3
T4   | 204   VDD_TEMP   T4
U2   | 205   VSYS_MON   U2
C3   | 206   WARMRSTN   C3
T1   | 207   XTAL_XI   T1
R1   | 208   XTAL_XO   R1
[Model Data]
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[End Model Data]
[End Package Model]
| Models and submodels in the file (68): BC40D_H_PUPDOFF_5P_SC1_1P8 (I/O), BC40D_H_PD_ON_5P_!SC1_1P8 (I/O), BC40D_H_PD_ON_5P_SC1_1P8 (I/O), BC40D_H_PU_ON_5P_!SC1_1P8 (I/O), BC40D_H_PUPDOFF_5P_!SC1_1P8 (I/O), BC40D_H_PU_ON_5P_SC1_1P8 (I/O), BC40D_H_PUPDOFF_5P_SC1_3P3 (I/O), BC40D_H_PD_ON_5P_!SC1_3P3 (I/O), BC40D_H_PD_ON_5P_SC1_3P3 (I/O), BC40D_H_PU_ON_5P_!SC1_3P3 (I/O), BC40D_H_PUPDOFF_5P_!SC1_3P3 (I/O), BC40D_H_PU_ON_5P_SC1_3P3 (I/O), BC40D_H_PUPDOFF_10P_SC1_1P8 (I/O), BC40D_H_PD_ON_10P_!SC1_1P8 (I/O), BC40D_H_PD_ON_10P_SC1_1P8 (I/O), BC40D_H_PU_ON_10P_!SC1_1P8 (I/O), BC40D_H_PUPDOFF_10P_!SC1_1P8 (I/O), BC40D_H_PU_ON_10P_SC1_1P8 (I/O), BC40D_H_PUPDOFF_10P_SC1_3P3 (I/O), BC40D_H_PD_ON_10P_!SC1_3P3 (I/O), BC40D_H_PD_ON_10P_SC1_3P3 (I/O), BC40D_H_PU_ON_10P_!SC1_3P3 (I/O), BC40D_H_PUPDOFF_10P_!SC1_3P3 (I/O), BC40D_H_PU_ON_10P_SC1_3P3 (I/O), BC40D_V_PUPDOFF_5P_SC1_1P8 (I/O), BC40D_V_PD_ON_5P_!SC1_1P8 (I/O), BC40D_V_PD_ON_5P_SC1_1P8 (I/O), BC40D_V_PU_ON_5P_!SC1_1P8 (I/O), BC40D_V_PUPDOFF_5P_!SC1_1P8 (I/O), BC40D_V_PU_ON_5P_SC1_1P8 (I/O), BC40D_V_PUPDOFF_5P_SC1_3P3 (I/O), BC40D_V_PD_ON_5P_!SC1_3P3 (I/O), BC40D_V_PD_ON_5P_SC1_3P3 (I/O), BC40D_V_PU_ON_5P_!SC1_3P3 (I/O), BC40D_V_PUPDOFF_5P_!SC1_3P3 (I/O), BC40D_V_PU_ON_5P_SC1_3P3 (I/O), BC40D_V_PUPDOFF_10P_SC1_1P8 (I/O), BC40D_V_PD_ON_10P_!SC1_1P8 (I/O), BC40D_V_PD_ON_10P_SC1_1P8 (I/O), BC40D_V_PU_ON_10P_!SC1_1P8 (I/O), BC40D_V_PUPDOFF_10P_!SC1_1P8 (I/O), BC40D_V_PU_ON_10P_SC1_1P8 (I/O), BC40D_V_PUPDOFF_10P_SC1_3P3 (I/O), BC40D_V_PD_ON_10P_!SC1_3P3 (I/O), BC40D_V_PD_ON_10P_SC1_3P3 (I/O), BC40D_V_PU_ON_10P_!SC1_3P3 (I/O), BC40D_V_PUPDOFF_10P_!SC1_3P3 (I/O), BC40D_V_PU_ON_10P_SC1_3P3 (I/O), BI2C1833_NORAML_5P_1P8 (I/O_open_drain), BI2C1833_NORAML_5P_3P3 (I/O_open_drain), BI2C1833_NORAML_10P_1P8 (I/O_open_drain), BI2C1833_NORAML_10P_3P3 (I/O_open_drain), IHHV_NORAML_5P_1P8 (Input), IHHV_NORAML_5P_3P3 (Input), IHHV_NORAML_10P_1P8 (Input), IHHV_NORAML_10P_3P3 (Input), IQ_SSDHH_PD_ON_5P_1P8 (Input), IQ_SSDHH_PU_ON_5P_1P8 (Input), IQ_SSDHH_PUPDOFF_5P_1P8 (Input), IQ_SSDHH_PD_ON_5P_3P3 (Input), IQ_SSDHH_PU_ON_5P_3P3 (Input), IQ_SSDHH_PUPDOFF_5P_3P3 (Input), IQ_SSDHH_PD_ON_10P_1P8 (Input), IQ_SSDHH_PU_ON_10P_1P8 (Input), IQ_SSDHH_PUPDOFF_10P_1P8 (Input), IQ_SSDHH_PD_ON_10P_3P3 (Input), IQ_SSDHH_PU_ON_10P_3P3 (Input), IQ_SSDHH_PUPDOFF_10P_3P3 (Input)
